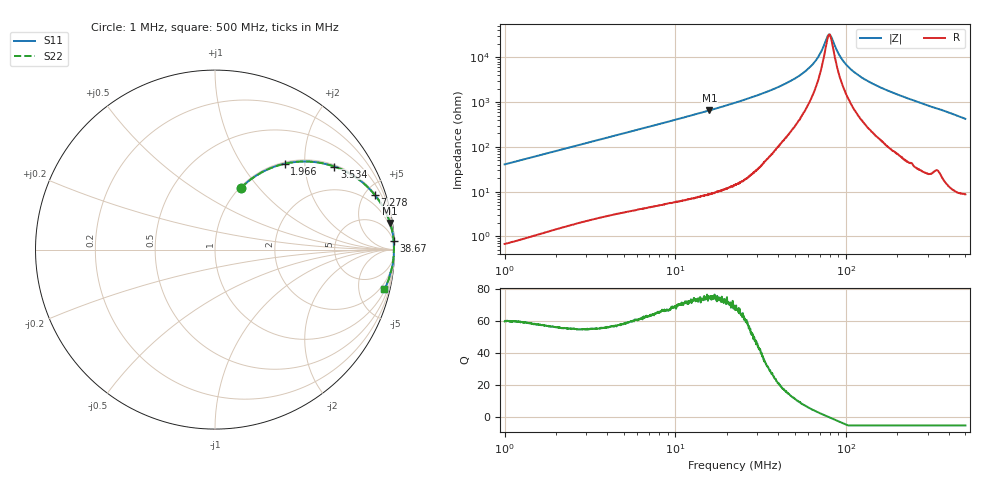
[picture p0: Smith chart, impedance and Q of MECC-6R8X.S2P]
!s-Parameter Generated by FASTRON Sdn. Bhd.
!FASTRON P/N : MECC-6R8X
!Keysight Technologies,E4991B,MY54100416,A.01.15
!Date: Mon Mar 16 15:12:21 2026
!Version  : Rev00 Mon Mar 16 15:12:21 2026
!Data & Calibration Information:
!PortZ  Port1:50+j0  Port2:50+j0
!When reading, reference impedance value at option line is always used.
!Remarks : This data is being provided solely for informational purposes.
!Freq	S11	S21	S12	S22
# Hz S dB R 50
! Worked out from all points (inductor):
!   1601 points, 1 MHz to 500 MHz, reference 50 ohm
!   read as one part in series: L = 6.45 uH near 1.032 MHz
!   highest Q = 74.9 at 15.83 MHz (marker M1), where L = 6.56 uH
!   self-resonance near 79.63 MHz
!   S11 on the Smith chart (normalised r, x): 1 MHz: 1.01, +0.81; 1.966 MHz: 1.03, +1.59; 3.534 MHz: 1.05, +2.84; 7.278 MHz: 1.09, +5.84; 38.67 MHz: 3, +41; 500 MHz: 1.17, -8.45
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1000000  -8.53 67.1  -0.71 -22.0  -0.71 -22.0  -8.53 67.1
1965681  -4.20 50.9  -2.20 -38.1  -2.20 -38.1  -4.20 50.9
2820919  -2.57 40.9  -3.68 -48.0  -3.68 -48.0  -2.57 40.9
3533689  -1.82 34.8  -4.87 -54.1  -4.87 -54.1  -1.82 34.8
5071144  -1.00 26.0  -7.16 -63.0  -7.16 -63.0  -1.00 26.0
7277522  -0.52 18.8  -9.83 -70.3  -9.83 -70.3  -0.52 18.8
7957584  -0.44 17.3  -10.53 -71.8  -10.53 -71.8  -0.44 17.3
1.58254e7  -0.12 8.7  -16.41 -80.5  -16.41 -80.5  -0.12 8.7
2.236068e7  -0.06 5.9  -19.75 -83.3  -19.75 -83.3  -0.06 5.9
3.866622e7  -0.03 2.8  -26.23 -84.8  -26.23 -84.8  -0.03 2.8
5.154174e7  -0.03 1.6  -31.10 -83.0  -31.10 -83.0  -0.03 1.6
6.307767e7  -0.03 0.8  -36.52 -77.9  -36.52 -77.9  -0.03 0.8
7.005203e7  -0.03 0.5  -41.29 -69.1  -41.29 -69.1  -0.03 0.5
7.779754e7  -0.03 0.1  -49.25 -27.1  -49.25 -27.1  -0.03 0.1
8.02529e7  -0.03 -0.0  -50.23 6.3  -50.23 6.3  -0.03 -0.0
8.246482e7  -0.03 -0.1  -48.71 32.8  -48.71 32.8  -0.03 -0.1
9.301677e7  -0.03 -0.5  -40.01 71.3  -40.01 71.3  -0.03 -0.5
1.057371e8  -0.03 -1.0  -34.95 78.9  -34.95 78.9  -0.03 -1.0
1.299065e8  -0.03 -1.8  -29.99 82.6  -29.99 82.6  -0.03 -1.8
1.77937e8  -0.04 -3.2  -24.99 83.7  -24.99 83.7  -0.04 -3.2
3.497673e8  -0.14 -8.1  -17.02 79.7  -17.02 79.7  -0.14 -8.1
5e8  -0.28 -13.2  -12.80 75.6  -12.80 75.6  -0.28 -13.2
